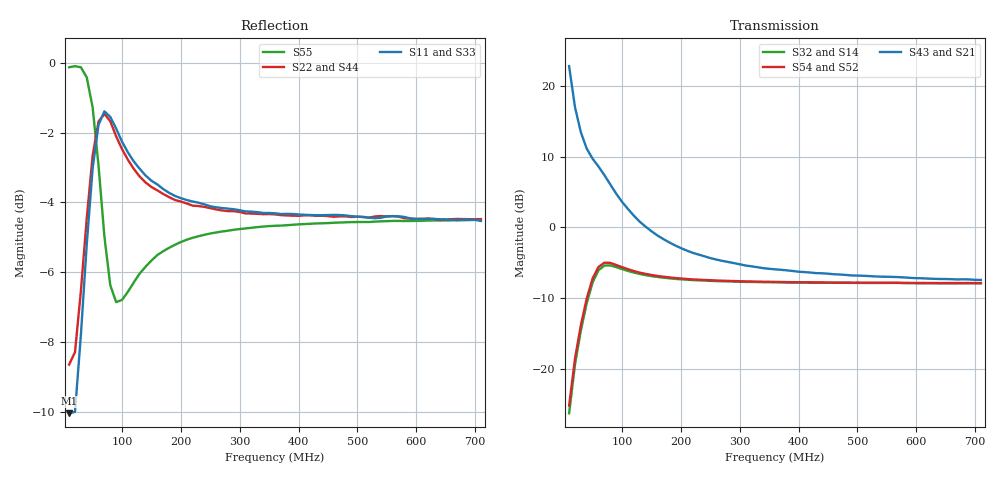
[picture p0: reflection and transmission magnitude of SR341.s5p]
!  POLYFET RF DEVICES
!  SR341  (Each side)
!  S PARAMETERS
!  VDS=50V, IDQ=400mA
!AWR Design Environment (2053) Wed Feb 04 15:55:41 2004
!freq-unit  param-type  data-format  keyword  impedance-ohms
# MHz  S  MA  R  50
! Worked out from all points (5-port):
!   71 points, 10 MHz to 710 MHz, reference 50 ohm
!   strongest paths, dB at 10 MHz, 180 MHz, 360 MHz, 540 MHz, 710 MHz:
!     S43: 22.8, -2.1, -5.9, -7.0, -7.4
!     S21: 22.8, -2.1, -5.9, -7.0, -7.4
!     S54: -25.2, -7.1, -7.7, -7.8, -7.9
!     S52: -25.2, -7.1, -7.7, -7.8, -7.9
!     S32: -26.3, -7.2, -7.8, -7.9, -7.9
!     S14: -26.3, -7.2, -7.8, -7.9, -7.9
!   lowest |S11| = -10.0 dB at 10 MHz (marker M1), VSWR 1.92, Z = 54.6 - j34.3 ohm
!   |S11| at or under -10 dB: start of sweep to 20.03 MHz
